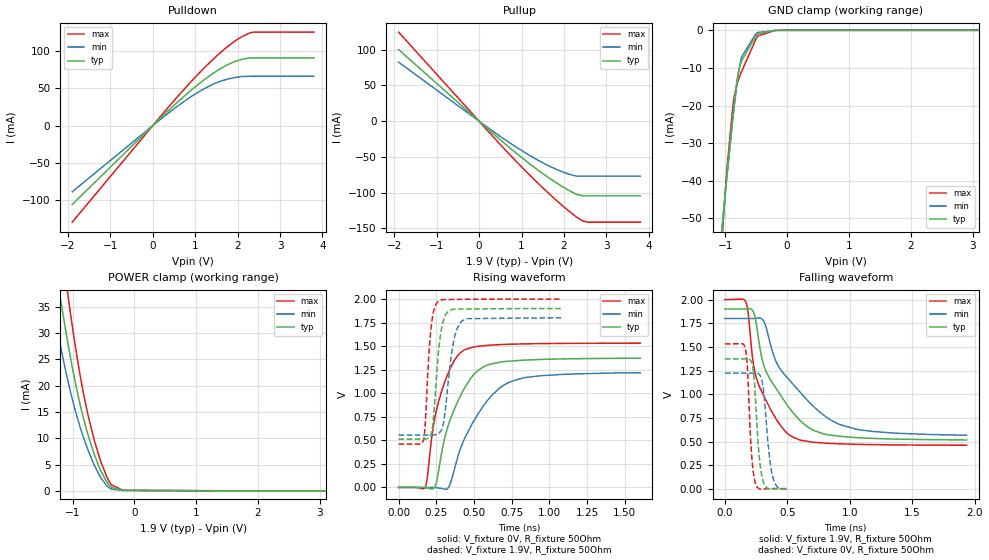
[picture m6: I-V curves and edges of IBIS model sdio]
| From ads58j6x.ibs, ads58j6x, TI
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|   sdio Model
[Model]   sdio
Model_type   I/O
Polarity   Non-Inverting
Enable   Active-High
Vinl = 0.4
Vinh = 1.2
Vmeas = 0.6
Vref = 0
Cref = 10pF
Rref = 50
|   typ   min   max
|   (nom PVT)   (fast PVT)   (slow PVT)
|Average
C_comp   5.599e-13   5.331e-13   5.951e-13
| Where nom  PVT is Nominal Process, 1.9V, 25C
|   Fast PVT is Strong Process,  2V, -40C
|   Slow PVT is Weak Process,   1.8V, 85C
[Voltage Range]   1.9   1.8   2
|Ambient Temperature   25   85   -40
|Junction Temperature
[Temperature Range]   25   85   -40
[Pullup Reference]   1.9   1.8   2
[Pulldown Reference]   0   0   0
[Power Clamp Reference]   1.9   1.8   2
[GND Clamp Reference]   0   0   0
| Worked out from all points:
|   slope of the pulldown table from 0 to 0.285 V, typ, clamps not added: 18.2 ohm
|   slope of the pullup table from 0 to 0.285 V, typ, clamps not added: 18.9 ohm
|   GND clamp passes 1 mA (typ) near -0.47 V on its own axis
|   POWER clamp passes 1 mA (typ) near -0.40 V on its own axis
|   falling waveform, V_fixture 1.9V, R_fixture 50Ohm: 20-80 % time 287ps typ, 399ps min, 198ps max; typ from 1.9 V to 0.516 V
|   rising waveform, V_fixture 0V, R_fixture 50Ohm: 20-80 % time 178ps typ, 237ps min, 128ps max; typ from 0 V to 1.37 V
|   rising waveform, V_fixture 1.9V, R_fixture 50Ohm: 20-80 % time 44.1ps typ, 55.8ps min, 35.2ps max; typ from 0.512 V to 1.9 V
|   falling waveform, V_fixture 0V, R_fixture 50Ohm: 20-80 % time 42.2ps typ, 51.8ps min, 34.5ps max; typ from 1.37 V to 0.003 V
[Pulldown]
|   Voltage   I(typ)   I(min)   I(max)
-1.9V     -105.8mA   -88.82mA   -129.6mA
36.1mV    2.014mA    1.688mA    2.469mA
719mV     38.3mA     31.58mA    47.47mA
1.158V    59.08mA    47.76mA    74.14mA
1.39V     68.82mA    54.67mA    87.2mA
1.604V    76.64mA    59.57mA    98.32mA
1.824V    83.23mA    63.06mA    108.6mA
2.092V    88.76mA    65.77mA    118.9mA
2.35V     90.7mA     66.08mA    125.1mA
3.8V      90.7mA     66.08mA    125.4mA
[GND Clamp]
|   Voltage   I(typ)   I(min)   I(max)
-1.9V     -341mA     -316.1mA   -362.1mA
-1.044V   -52.61mA   -51.19mA   -54.1mA
-1.024V   -48.54mA   -47.71mA   -48.93mA
-974.7mV  -39.21mA   -39.39mA   -37.53mA
-876mV    -22.52mA   -23.71mA   -20.21mA
-855mV    -19.35mA   -20.59mA   -17.69mA
-789.4mV  -11.43mA   -11.94mA   -13.36mA
-735.3mV  -8.162mA   -7.125mA   -11.01mA
-506.8mV  -1.554mA   -1mA       -2.486mA
-468mV    -904.8uA   -571.5uA   -1.484mA
-190mV    -10.03uA   -8.658uA   -11.85uA
3.8V      0A         0A         0A
[Pullup]
|   Voltage   I(typ)   I(min)   I(max)
-1.9V     100.4mA    82.75mA    124.8mA
197mV     -10.51mA   -8.617mA   -13.12mA
946.2mV   -48.19mA   -38.97mA   -60.66mA
1.642V    -79.28mA   -62.54mA   -101.2mA
1.977V    -92.16mA   -71.24mA   -118.9mA
2.281V    -102mA     -76.79mA   -133.5mA
2.44V     -104.4mA   -76.99mA   -139.6mA
2.57V     -104.5mA   -76.99mA   -141.4mA
3.8V      -104.5mA   -76.99mA   -141.4mA
[POWER Clamp]
|   Voltage   I(typ)   I(min)   I(max)
-1.9V     99.86mA    82.86mA    122.3mA
-1.393V   51.91mA    40.73mA    67.18mA
-1.22V    38.35mA    29.09mA    50.41mA
-1.18V    35.43mA    26.7mA     46.7mA
-1.066V   27.48mA    20.47mA    36.5mA
-914mV    18.33mA    13.57mA    24.52mA
-828mV    14.04mA    10.35mA    18.83mA
-740mV    10.29mA    7.487mA    13.94mA
-558mV    4.243mA    2.819mA    6.139mA
-385.7mV  849.6uA    434.6uA    1.411mA
-174mV    105.4uA    85.75uA    135uA
3.8V      0A         0A         0A
[Ramp]
R_load = 50
|   typ   min   max
dV/dt_r   0.823741/1.77835e-10 0.733552/2.39605e-10   0.918903/1.27993e-10
dV/dt_f   0.8326/2.8887e-10   0.746389/4.0478e-10   0.924331/1.9803e-10
[Falling Waveform]
V_fixture = 1.9V
V_fixture_min = 1.8V
V_fixture_max = 2V
R_fixture = 50Ohm
|   Time   V(typ)   V(min)   V(max)
0s        1.9V       1.8V       2V
168ps     1.9V       1.8V       1.974V
230ps     1.865V     1.8V       1.307V
268ps     1.597V     1.807V     1.11V
328ps     1.244V     1.719V     938mV
406ps     1.068V     1.354V     746.7mV
520ps     847.5mV    1.143V     566.2mV
694ps     629.1mV    890.7mV    494.5mV
912ps     555.9mV    682.9mV    476mV
1.934ns   516.3mV    566.3mV    460.7mV
[Rising Waveform]
V_fixture = 0V
V_fixture_min = 0V
V_fixture_max = 0V
R_fixture = 50Ohm
|   Time   V(typ)   V(min)   V(max)
0s        78.87nV    85.23nV    151nV
178ps     -2.88mV    30.71uV    3.905mV
236ps     -7.163mV   -1.253mV   700.2mV
262ps     143.4mV    -5.423mV   891.8mV
292ps     422.5mV    -13.67mV   1.054V
330ps     661.4mV    -2.972mV   1.217V
436ps     1.051V     513.2mV    1.459V
590ps     1.301V     925mV      1.508V
762ps     1.344V     1.134V     1.521V
1.602ns   1.371V     1.218V     1.531V
[Rising Waveform]
V_fixture = 1.9V
V_fixture_min = 1.8V
V_fixture_max = 2V
R_fixture = 50Ohm
|   Time   V(typ)   V(min)   V(max)
0s        512.3mV    555.9mV    459.4mV
164ps     512.1mV    555.9mV    497.3mV
176ps     512.8mV    556mV      653.3mV
202ps     529.3mV    555.9mV    1.437V
222ps     605.4mV    555.9mV    1.776V
262ps     1.392V     569.1mV    1.974V
314ps     1.839V     874.7mV    1.995V
364ps     1.892V     1.546V     1.996V
422ps     1.894V     1.769V     1.997V
1.078ns   1.899V     1.799V     2V
[Falling Waveform]
V_fixture = 0V
V_fixture_min = 0V
V_fixture_max = 0V
R_fixture = 50Ohm
|   Time   V(typ)   V(min)   V(max)
0s        1.373V     1.223V     1.532V
164ps     1.373V     1.223V     1.482V
180ps     1.375V     1.223V     1.287V
222ps     1.295V     1.223V     237.4mV
252ps     788.7mV    1.224V     33.73mV
276ps     328.4mV    1.208V     -201.7uV
312ps     57.63mV    1.009V     -2.874mV
360ps     -2.405mV   300.1mV    1.906mV
388ps     -2.14mV    102.9mV    2.62mV
500ps     2.558mV    -3.453mV   1.044mV
